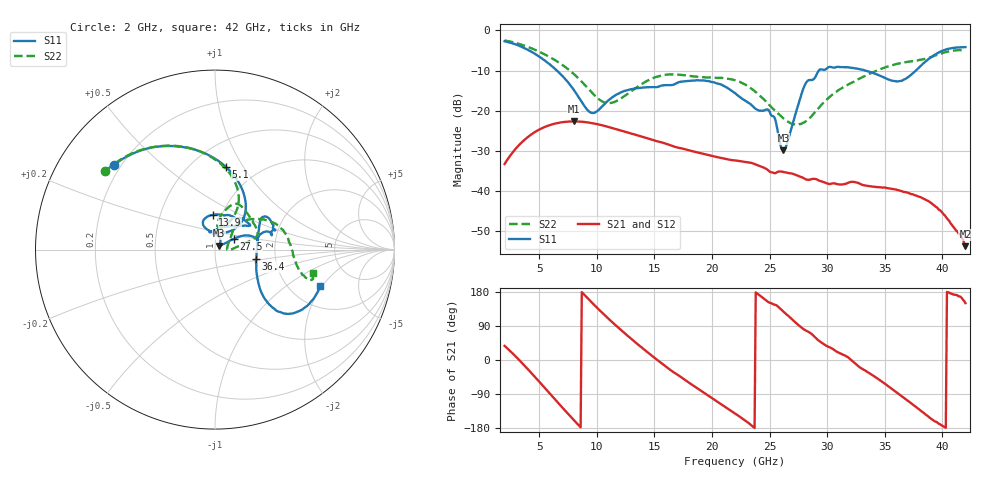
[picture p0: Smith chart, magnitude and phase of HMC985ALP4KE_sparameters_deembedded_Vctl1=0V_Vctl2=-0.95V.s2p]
!s2p File: Measurements: S11, S21, S12, S22
# GHz S dB R 50.0
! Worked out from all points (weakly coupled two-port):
!   401 points, 2 GHz to 42 GHz, reference 50 ohm
!   highest |S21| = -22.64 dB at 8 GHz (marker M1); lowest = -53.7 dB at 42 GHz (marker M2)
!   lowest |S11| = -29.8 dB at 26.2 GHz (marker M3), VSWR 1.07, Z = 52.4 + j2.25 ohm
!   |S11| at or under -10 dB: 6.548 GHz to 29.27 GHz (22.72 GHz wide, 127 % of centre); 33.35 GHz to 37.69 GHz (4.345 GHz wide, 12.2 % of centre)
!   |S22| runs from -23.5 to -2.5 dB; largest |S21 - S12| = 0.00014
!   S11 on the Smith chart (normalised r, x): 2 GHz: 0.17, +0.35; 5.1 GHz: 0.72, +0.84; 13.9 GHz: 0.90, +0.36; 27.5 GHz: 1.22, +0.15; 36.4 GHz: 1.58, -0.17; 42 GHz: 2.91, -1.91
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2  -2.67 140.1  -33.27 37.2  -33.27 37.3  -2.48 144.6
3.5  -4.10 112.3  -27.83 -7.5  -27.83 -7.5  -3.57 120.2
5.1  -6.68 82.3  -24.53 -60.4  -24.54 -60.5  -5.41 95.8
8  -14.76 45.6  -22.64 -158.3  -22.65 -158.3  -10.81 63.0
8.7  -17.84 51.8  -22.73 179.1  -22.73 179.1  -12.76 60.7
9.7  -20.55 85.8  -23.12 147.8  -23.12 147.8  -15.83 64.1
11  -17.41 114.5  -24.01 109.4  -24.01 109.4  -18.10 79.0
13.9  -14.24 93.9  -26.42 32.9  -26.43 32.9  -13.32 77.1
15.4  -13.94 73.0  -27.68 -3.0  -27.69 -3.1  -11.36 68.3
19.4  -12.52 34.6  -30.84 -88.3  -30.85 -88.4  -11.67 36.0
22  -15.60 52.2  -32.38 -140.8  -32.39 -140.9  -12.40 17.0
25  -20.19 97.8  -35.13 151.2  -35.15 151.2  -18.62 6.2
26.2  -29.82 41.7  -35.22 127.6  -35.23 127.5  -21.88 -1.7
27.5  -18.41 29.7  -36.21 92.5  -36.19 92.3  -23.39 5.0
28.1  -13.36 20.7  -36.98 78.6  -37.01 78.4  -22.72 16.7
28.7  -12.31 12.8  -36.97 67.5  -36.97 67.4  -21.15 28.2
31  -9.08 23.3  -38.30 19.5  -38.32 19.4  -14.82 48.7
33.3  -9.96 34.4  -38.62 -27.7  -38.62 -27.8  -11.32 38.6
35.4  -12.27 12.3  -39.33 -71.5  -39.32 -71.2  -8.85 24.1
36.4  -12.57 -12.8  -39.97 -94.0  -39.99 -94.0  -8.08 16.2
39.5  -5.80 -43.3  -43.99 -163.4  -43.98 -164.3  -6.09 -14.6
42  -4.14 -19.0  -53.71 150.0  -53.56 151.4  -4.99 -13.5
